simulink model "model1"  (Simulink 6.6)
settings: Solver=VariableStepDiscrete  StartTime=0.0  StopTime=0.0  RelTol=1e-3
libraries: ltpda_library x1

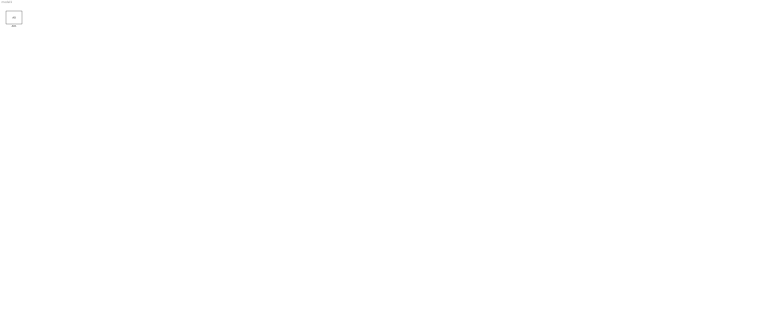
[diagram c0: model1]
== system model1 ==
  note: .
  AO1 : ltpda_library/Input/AO  Tag=input  SystemSampleTime=-1
